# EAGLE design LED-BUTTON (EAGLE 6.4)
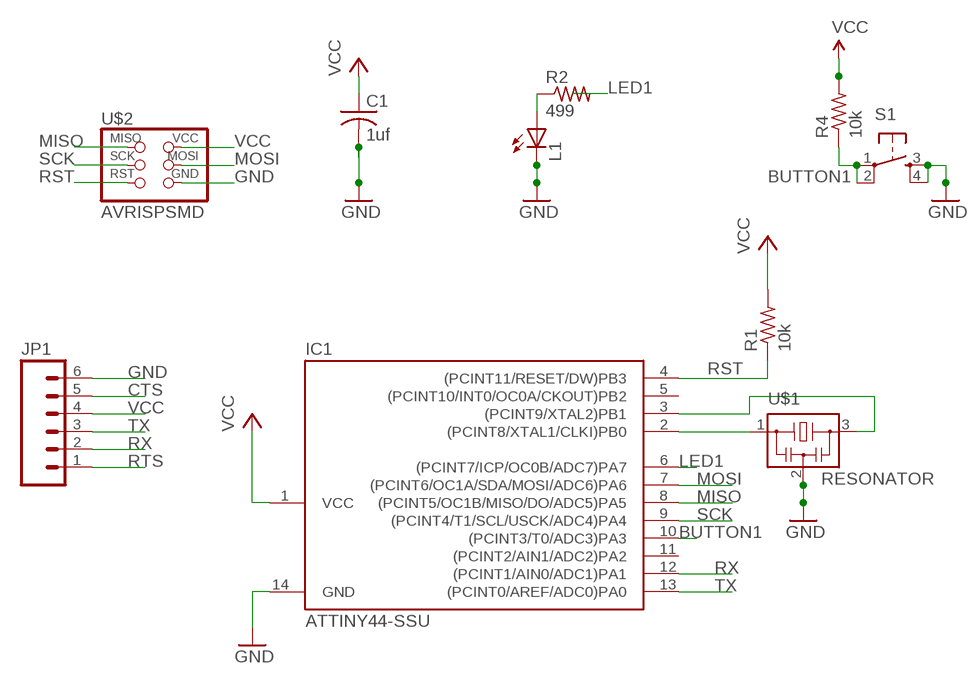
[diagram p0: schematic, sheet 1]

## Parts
C1  1uf  C-USC1206  [C1206]
IC1  ATTINY44-SSU  [SOIC14]
JP1  M06SMD  [1X06-SMD]
L1  LED1206  [1206]
R1  10k  R-US_R1206  [R1206]
R2  499  RESISTOR1206  [1206]
R4  10k  RESISTOR1206  [1206]
S1  6MM_SWITCH6MM_SWITCH  [6MM_SWITCH]
U$1  RESONATOR  [EFOBM]
U$2  AVRISPSMD  [2X03SMD]

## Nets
BUTTON1: IC1.10((PCINT3/T0/ADC3)PA3) R4.1 S1.1(P) S1.2(P1)
CTS: JP1.5
GND: C1.2 IC1.14(GND) JP1.6 L1.2(C) S1.3(S) S1.4(S1) U$1.2 U$2.6(GND)
LED1: IC1.6((PCINT7/ICP/OC0B/ADC7)PA7) R2.2
MISO: IC1.8((PCINT5/OC1B/MISO/DO/ADC5)PA5) U$2.1(MISO)
MOSI: IC1.7((PCINT6/OC1A/SDA/MOSI/ADC6)PA6) U$2.4(MOSI)
N$1: IC1.2((PCINT8/XTAL1/CLKI)PB0) U$1.1
N$2: IC1.3((PCINT9/XTAL2)PB1) U$1.3
N$3: L1.1(A) R2.1
RST: IC1.4((PCINT11/RESET/DW)PB3) R1.1 U$2.5(RST)
RTS: JP1.1
RX: IC1.12((PCINT1/AIN0/ADC1)PA1) JP1.2
SCK: IC1.9((PCINT4/T1/SCL/USCK/ADC4)PA4) U$2.3(SCK)
TX: IC1.13((PCINT0/AREF/ADC0)PA0) JP1.3
VCC: C1.1 IC1.1(VCC) JP1.4 R1.2 R4.2 U$2.2(VCC)
Unconnected: IC1.5((PCINT10/INT0/OC0A/CKOUT)PB2) IC1.11((PCINT2/AIN1/ADC2)PA2)

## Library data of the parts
C1 = rcl:C-US: CAPACITOR, American symbol
IC1 = fab:ATTINY44
JP1 = SparkFun:M06: Header 6 Standard 6-pin 0.1" header. Use with straight break away headers (SKU : PRT-00116), right angle break away headers (PRT-00553), swiss pins (PRT-00743), machine pins (PRT-00117), and female headers (PRT-00115). Molex polarized connector foot print use with SKU : PRT-08094 with associated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
L1 = 01_FAB_Hello:LED
R1 = resistor:R-US_: RESISTOR, American symbol
R2 R4 = 01_ng:RESISTOR
S1 = 01_fab:6MM_SWITCH: OMRON SWITCH
U$1 = fab:RESONATOR
U$2 = fab:AVRISP

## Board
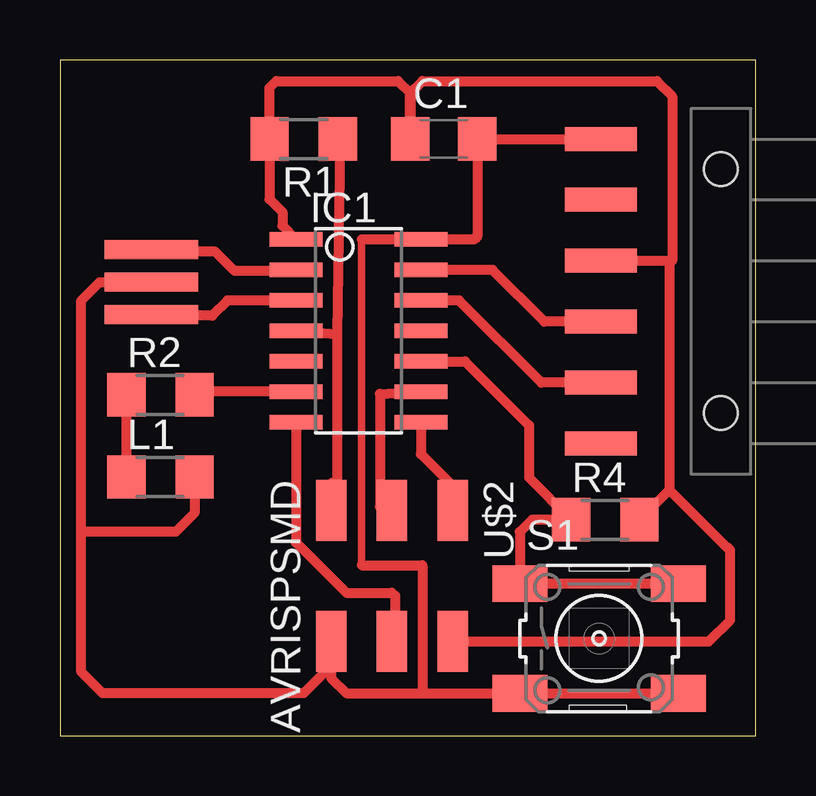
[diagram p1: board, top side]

Size 29.01 x 28.18 mm. Coordinates in mm from the lower left corner, seen from the top.
Outline: 0,0 29.01,0 29.01,28.18 0,28.18 0,0
Copper layers 1: Top 0.035mm
Design rules "ERP-1sided-10mil-16mill": minimum track width 10mil, minimum drill 24mil, track to track 16mil, track to pad 16mil, pad to pad 16mil, via to via 16mil, smd to smd 0mil, copper to edge 16mil, drill to drill 36mil, minimum pad ring 10mil, minimum via ring 8mil, stop-mask expansion 4mil, vias tented up to drill 0mil, thermal gap 10mil

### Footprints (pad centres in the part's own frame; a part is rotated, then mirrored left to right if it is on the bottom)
C1206 = smd 1.6 x 1.8: 1 -1.4,0; 2 1.4,0
SOIC14 = smd 0.61 x 2.21: 1 -3.81,-2.603; 2 -2.54,-2.603; 3 -1.27,-2.603; 4 0,-2.603; 5 1.27,-2.603; 6 2.54,-2.603; 7 3.81,-2.603; 8 3.81,2.603; 9 2.54,2.603; 10 1.27,2.603; 11 0,2.603; 12 -1.27,2.603; 13 -2.54,2.603; 14 -3.81,2.603
1X06-SMD = smd 1 x 3: 1 -6.35,5; 2 -3.81,5; 3 -1.27,5; 4 1.27,5; 5 3.81,5; 6 6.35,5 | hole 1.4: -5.08,0; 5.08,0
1206 = smd 1.6 x 1.803: 1 -1.422,0; 2 1.422,0
R1206 = smd 1.6 x 1.803: 1 -1.422,0; 2 1.422,0
6MM_SWITCH = smd 2.286 x 1.524: 1 -3.302,2.286; 2 3.302,2.286; 3 -3.302,-2.286; 4 3.302,-2.286
EFOBM = smd 0.8 x 3.9: 1 -1.35,0; 2 0,0; 3 1.35,0
2X03SMD = smd 2.54 x 1.27: 1 -2.54,2.54; 2 2.92,2.54; 3 -2.54,0; 4 2.92,0; 5 -2.54,-2.54; 6 2.92,-2.54

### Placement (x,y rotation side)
C1  16,24.89 0 top
IC1  12.45,16.89 270 top
JP1  27.56,18.54 90 top
L1  4.19,10.79 0 top
R1  10.16,24.89 180 top
R2  4.19,14.22 0 top
R4  22.73,9.02 0 top
S1  22.48,4.06 0 top
U$1  3.81,18.92 270 top
U$2  13.84,6.86 270 top

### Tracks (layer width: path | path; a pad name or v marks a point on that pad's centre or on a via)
BUTTON1
  Top 0.406: IC1.10 16.89,15.62 19.56,12.95 19.56,10.77 R4.1 19.68,9.02 19.18,8.51 S1.1 S1.2
GND
  Top 0.305: 12.57,20.7 12.57,7.11
  Top 0.406: JP1.6 C1.2 17.4,20.83 17.27,20.7 IC1.14 12.57,20.7 | S1.4 S1.3 15.11,1.78 | 12.57,7.11 15.11,7.11 15.11,1.78 | 0.89,8.38 0.89,2.67 1.78,1.78 10.16,1.78 11.3,2.92 U$2.6 11.3,2.41 11.94,1.78 15.11,1.78 | 0.89,8.38 0.89,18.16 1.65,18.92 U$1.2 | L1.2 5.61,9.3 4.83,8.51 1.02,8.51 0.89,8.38
LED1
  Top 0.406: IC1.6 5.74,14.35 R2.2
MISO
  Top 0.406: IC1.8 15.05,11.75 16.26,10.54 16.26,9.53 U$2.1
MOSI
  Top 0.406: IC1.7 9.84,8.06 11.94,5.97 13.84,5.97 13.97,5.84 13.97,4.7 14.1,4.57 14.1,4.19 U$2.4
N$1
  Top 0.406: IC1.2 9.8,19.38 7.29,19.38 6.48,20.19 3.89,20.19 U$1.1
N$2
  Top 0.406: IC1.3 6.99,18.16 6.35,17.53 3.86,17.53 U$1.3
N$3
  Top 0.406: R2.1 L1.1
RST
  Top 0.406: R1.1 11.68,24.77 11.56,16.76 | IC1.4 11.56,16.76 | 11.56,16.76 11.56,10.54 11.3,10.54 U$2.5
RX
  Top 0.406: 23.11,14.73 JP1.2 20.07,14.73 16.64,18.16 IC1.12
SCK
  Top 0.406: 13.46,9.53 U$2.3 13.34,9.56 13.34,14.26 IC1.9
TX
  Top 0.406: JP1.3 20.19,17.27 18.03,19.43 IC1.13
VCC
  Top 0.406: 25.4,19.81 25.53,19.81 25.53,26.67 24.89,27.3 15.11,27.3 14.6,26.79 C1.1 14.61,26.8 14.1,27.3 9.02,27.3 8.74,27.03 R1.2 8.74,22.38 9.27,21.84 9.27,21.27 IC1.1 | JP1.4 25.4,19.81 | 25.4,19.81 25.4,10.26 | 25.4,10.26 R4.2 | U$2.2 27.05,3.94 27.94,4.83 27.94,7.75 27.81,7.87 27.79,7.87 25.4,10.26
